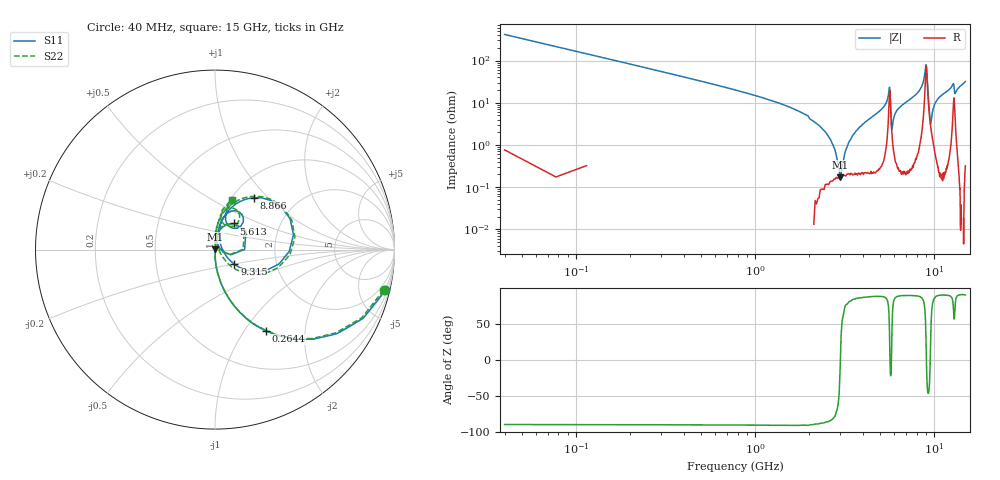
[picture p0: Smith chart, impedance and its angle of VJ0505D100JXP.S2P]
! VJ0505D100JXP
! MLCC placed on 25 mil thick microstrip substrate in series configuraton.
! DATE 06/29/2018  08:59
! CORRECTED  DATA
# GHz  S  MA  R  50.00
!  FREQ  S11M  S11A  S21M  S21A  S12M  S12A  S22M  S22A
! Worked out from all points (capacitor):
!   401 points, 40 MHz to 15 GHz, reference 50 ohm
!   read as one part in series: C = 9.54 pF near 114.8 MHz
!   lowest |Z| = 173 mohm at 2.995 GHz (marker M1)
!   series resonance near 3.004 GHz, so ESL is about 290 pH
!   S11 on the Smith chart (normalised r, x): 40 MHz: 0.89, -8.38; 264.4 MHz: 0.99, -1.26; 5.613 GHz: 1.18, +0.36; 8.866 GHz: 1.25, +0.83; 9.315 GHz: 1.22, -0.20; 15 GHz: 1.02, +0.62
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0.04  0.9757 -13.5  0.2334 76.4  0.2337 76.6  0.9665 -13.5
0.2644  0.5328 -58.1  0.8474 32.1  0.8481 32.2  0.5284 -58.0
0.7506  0.2053 -79.0  0.98 11.8  0.9804 11.9  0.204 -78.9
2.5458  0.01484 -85.3  0.9974 1.1  0.9981 1.1  0.0146 -91.0
2.7328  0.007425 -79.0  0.9972 0.7  0.9979 0.7  0.007091 -93.4
2.8824  0.002271 -47.1  0.9971 0.4  0.9976 0.4  0.001448 -102.5
2.9946  0.002807 45.3  0.9972 0.1  0.998 0.2  0.002205 92.9
3.1442  0.007323 72.1  0.9967 -0.2  0.9976 -0.1  0.007165 92.0
3.4434  0.01662 79.0  0.9967 -0.7  0.997 -0.6  0.01639 90.9
5.0516  0.07063 81.8  0.9932 -3.7  0.9938 -3.6  0.0693 87.5
5.6126  0.1803 53.8  0.9072 -8.8  0.9077 -8.7  0.1753 56.2
5.837  0.02763 43.2  0.9819 -0.7  0.9826 -0.7  0.02267 57.0
6.2484  0.0713 81.2  0.9932 -3.7  0.994 -3.6  0.07081 88.3
7.52  0.1292 79.1  0.9872 -7.2  0.9884 -7.2  0.1318 84.8
8.8664  0.3613 53.1  0.8332 -20.5  0.834 -20.5  0.3688 53.7
9.0908  0.4136 -1.5  0.5839 2.0  0.5844 2.0  0.4183 -3.9
9.3152  0.1359 -37.1  0.9036 5.5  0.9045 5.5  0.1286 -46.3
9.577  0.03868 17.8  0.9703 -0.6  0.9709 -0.6  0.02045 29.2
10.0258  0.08424 74.8  0.9861 -4.7  0.9872 -4.7  0.08421 85.7
12.5316  0.2182 70.2  0.9606 -13.3  0.9615 -13.3  0.225 76.7
13.13  0.152 58.9  0.9428 -8.9  0.9441 -8.9  0.1488 69.7
15  0.292 71.5  0.9507 -18.3  0.9512 -18.3  0.2931 71.4
